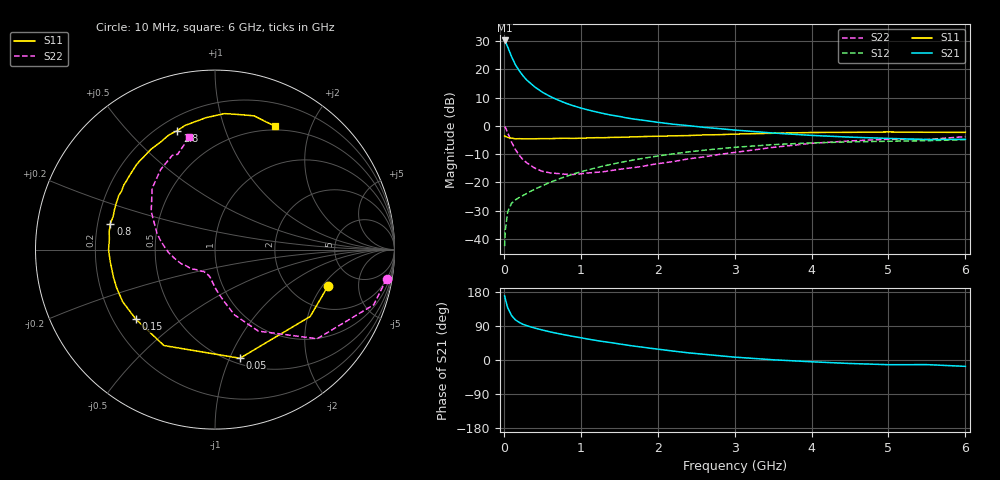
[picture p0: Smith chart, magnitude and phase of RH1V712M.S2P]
! SIEMENS Small Signal Semiconductors
! BFR106
! Si NPN RF Bipolar Junction Transistor in SOT23
! VCE = 1.75 V  IC = 12 mA
! Common Emitter S-Parameters:  August  1996
# GHz  S  MA  R  50
!  f  S11  S21  S12  S22
! GHz  MAG  ANG  MAG  ANG  MAG  ANG  MAG  ANG
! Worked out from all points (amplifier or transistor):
!   36 points, 10 MHz to 6 GHz, reference 50 ohm
!   highest |S21| = 30.2 dB at 10 MHz (marker M1)
!   |S21| within 3 dB of that: start of sweep to 60.19 MHz
!   unconditionally stable (mu >= 1): 436.4 MHz to 2.48 GHz; 4.646 GHz to end of sweep
!   at 250 MHz: K = 0.78, MSG = 21.2 dB, |S12| = -24.7 dB
!   at 1.4 GHz: K = 1.10, MAG = 6.8 dB, |S12| = -13.6 dB
!   at 6 GHz: K = 1.02, MAG = -0.8 dB, |S12| = -4.9 dB
!   S11 on the Smith chart (normalised r, x): 10 MHz: 3.12, -2.28; 50 MHz: 0.55, -1.09; 150 MHz: 0.29, -0.35; 800 MHz: 0.25, +0.12; 2.8 GHz: 0.27, +0.70; 6 GHz: 0.45, +1.50
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0.01  0.6611 -18.1  32.31 169.4  0.0074 83.1  0.9702 -9.7
0.02  0.6482 -35.1  30.83 160.5  0.0144 75.6  0.9358 -19.2
0.05  0.6211 -77.1  24.77 137.9  0.03 58.9  0.7555 -41.1
0.1  0.6054 -118.0  16.76 117.4  0.0425 47.5  0.5142 -62.0
0.15  0.5873 -138.6  12.05 105.9  0.0488 44.6  0.3804 -73.3
0.2  0.5908 -150.6  9.409 99.3  0.0538 45.5  0.302 -79.2
0.25  0.5878 -158.8  7.616 94.1  0.0584 47.1  0.2494 -84.9
0.3  0.5864 -164.7  6.405 90.4  0.0639 49.5  0.2201 -88.7
0.4  0.5877 -173.6  4.887 84.4  0.0752 53.0  0.1786 -95.0
0.5  0.5931 180.0  3.932 79.2  0.0866 55.6  0.1563 -100.0
0.6  0.5913 174.5  3.31 74.3  0.0996 57.3  0.1467 -104.4
0.7  0.598 170.3  2.867 70.0  0.1121 58.5  0.1428 -109.1
0.8  0.6009 166.0  2.523 66.0  0.126 59.0  0.1387 -113.8
1.1  0.6085 154.3  1.896 55.0  0.1665 58.9  0.1463 -125.9
1.3  0.6142 147.9  1.639 48.4  0.1946 57.5  0.1539 -133.9
1.6  0.6305 138.9  1.372 39.3  0.2362 54.8  0.1761 -145.6
2.2  0.6633 122.5  1.066 23.6  0.3183 47.1  0.2323 -168.3
2.8  0.6955 107.6  0.889 11.3  0.3921 37.7  0.311 169.8
3.5  0.7364 94.0  0.744 0.6  0.4636 26.3  0.4143 149.1
4.5  0.7651 79.3  0.629 -9.2  0.5177 10.7  0.5389 124.2
5.5  0.7662 68.2  0.571 -12.2  0.5436 1.0  0.5699 111.5
6  0.7653 64.2  0.575 -16.8  0.5688 -6.1  0.6428 102.8
